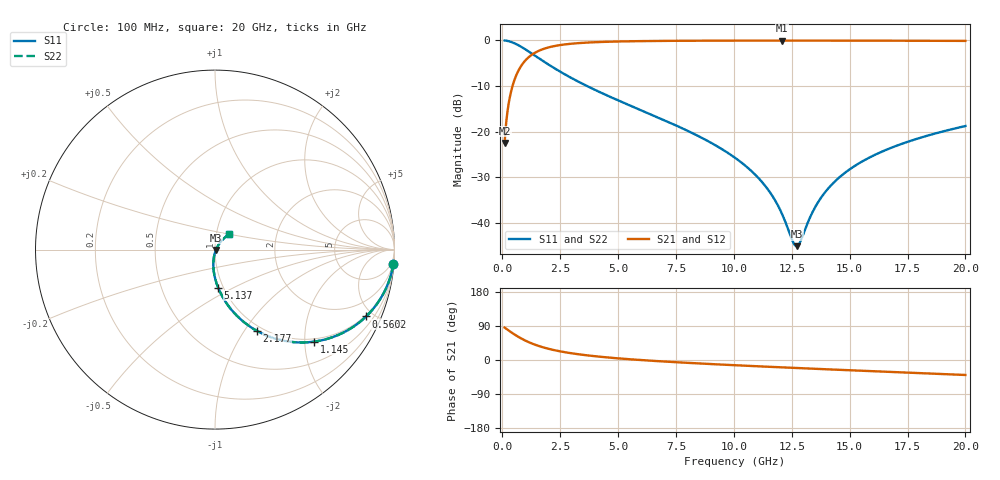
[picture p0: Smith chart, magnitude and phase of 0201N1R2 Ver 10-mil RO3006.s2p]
# GHz S MA R 50
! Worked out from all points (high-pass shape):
!   1601 points, 100 MHz to 20 GHz, reference 50 ohm
!   highest |S21| = -0.05 dB at 12.06 GHz (marker M1); lowest = -22.5 dB at 100 MHz (marker M2)
!   |S21| within 3 dB of the highest: 1.304 GHz to end of sweep
!   lowest |S11| = -45.1 dB at 12.71 GHz (marker M3), VSWR 1.01, Z = 50.5 - j0.205 ohm
!   |S11| at or under -10 dB: 3.659 GHz to end of sweep
!   |S22| runs from -45.1 to 0.0 dB; largest |S21 - S12| = 0
!   S11 on the Smith chart (normalised r, x): 100 MHz: 1, -26; 560.2 MHz: 0.93, -4.55; 1.145 GHz: 0.93, -2.21; 2.177 GHz: 0.93, -1.14; 5.137 GHz: 0.95, -0.42; 20 GHz: 1.15, +0.20
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0.1  0.9972 -4.5  0.07522 85.5  0.07522 85.5  0.9972 -4.5
0.3114375  0.9733 -13.7  0.2288 76.2  0.2288 76.2  0.9733 -13.7
0.5601875  0.9205 -23.9  0.3897 66.1  0.3897 66.1  0.9205 -23.9
0.821375  0.8485 -33.2  0.5278 56.7  0.5278 56.7  0.8485 -33.2
1.14475  0.7535 -42.9  0.6556 47.0  0.6556 47.0  0.7535 -42.9
1.629813  0.6241 -53.9  0.779 35.9  0.779 35.9  0.6241 -53.9
2.177062  0.5085 -62.8  0.8583 26.9  0.8583 26.9  0.5085 -62.8
3.420812  0.339 -75.4  0.9374 14.1  0.9374 14.1  0.339 -75.4
5.137187  0.2129 -85.3  0.973 3.7  0.973 3.7  0.2129 -85.3
6.741625  0.1425 -91.3  0.9853 -3.1  0.9853 -3.1  0.1425 -91.3
8.694313  0.08364 -96.4  0.9915 -9.7  0.9915 -9.7  0.08364 -96.4
10.05  0.05185 -98.2  0.9933 -13.8  0.9933 -13.8  0.05185 -98.2
11.25644  0.02739 -96.0  0.994 -17.2  0.994 -17.2  0.02739 -96.0
12.06488  0.01284 -84.2  0.9942 -19.4  0.9942 -19.4  0.01284 -84.2
12.5375  0.006357 -49.8  0.9941 -20.7  0.9941 -20.7  0.006357 -49.8
12.71162  0.005586 -21.3  0.9941 -21.1  0.9941 -21.1  0.005586 -21.3
12.87331  0.006286 5.1  0.9941 -21.6  0.9941 -21.6  0.006286 5.1
13.37081  0.01275 40.5  0.9939 -22.9  0.9939 -22.9  0.01275 40.5
13.90563  0.0212 49.9  0.9936 -24.3  0.9936 -24.3  0.0212 49.9
14.61456  0.03257 53.4  0.9932 -26.1  0.9932 -26.1  0.03257 53.4
16.69162  0.06507 53.1  0.9912 -31.3  0.9912 -31.3  0.06507 53.1
20  0.1154 47.1  0.986 -39.5  0.986 -39.5  0.1154 47.1
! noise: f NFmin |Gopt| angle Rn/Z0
0.1  0.0009902  0.9596  0.8711  0.005529
2.301  0.005362  0.8263  4.448  0.006482
4.515  0.008286  0.7845  8.009  0.00786
6.729  0.01081  0.7577  11.58  0.008935
8.943  0.01311  0.7381  15.14  0.009848
11.14  0.01527  0.723  18.66  0.01065
13.36  0.01735  0.7108  22.16  0.01139
15.57  0.01936  0.701  25.63  0.01208
17.79  0.02134  0.693  29.05  0.01272
20  0.02329  0.6865  32.43  0.01334
